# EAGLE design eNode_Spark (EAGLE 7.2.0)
REV: V3.3

## Sheet 1 of 4: Power & MCU
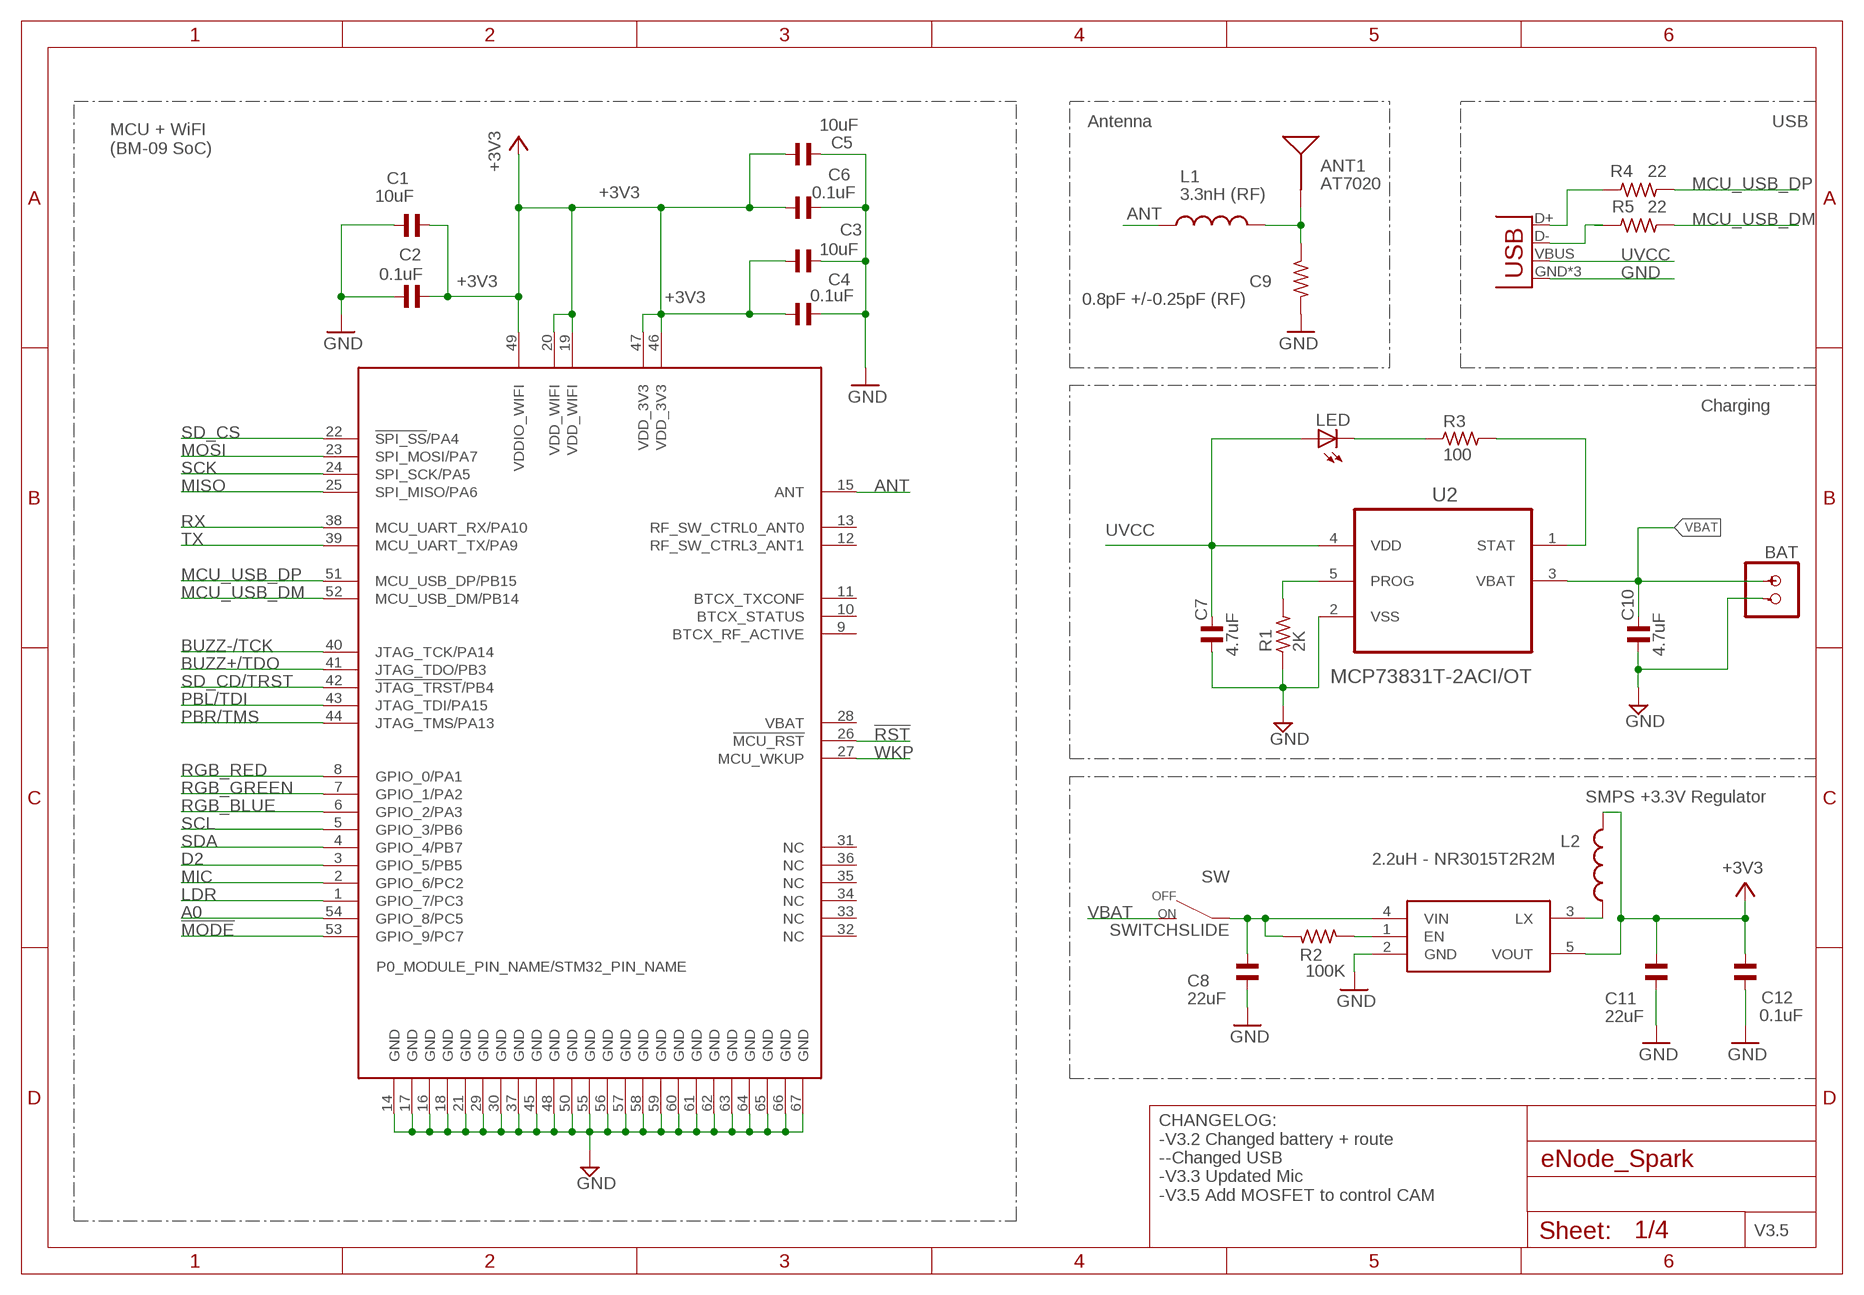
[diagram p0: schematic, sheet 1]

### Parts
ANT1  AT7020  [AT7020]
BAT  BATTERYSMT  [JST-2-SMD]
C1  10uF  C_0402  [C0402]
C2  0.1uF  C_0402  [C0402]
C3  10uF  C_0402  [C0402]
C4  0.1uF  C_0402  [C0402]
C5  10uF  C_0402  [C0402]
C6  0.1uF  C_0402  [C0402]
C7  4.7uF  C_0402  [C0402]
C8  22uF  C_0603  [C0603]
C9  0.8pF +/-0.25pF (RF)  R-US_  [R0402_B]
C10  4.7uF  C_0402  [C0402]
C11  22uF  C_0603  [C0603]
C12  0.1uF  C_0402  [C0402]
JP1  USBUSB-MICROB-SLOT-HOLE  [USB-MICROB-SLOT-HOLE]
L1  3.3nH (RF)  INDUCTOR  [L0402_B]
L2  2.2uH - NR3015T2R2M  INDUCTORB  [INDUCTOR-NR3015]
LED  LED  [SMARTLED-TTW]
R1  2K  R_0603  [R0603]
R2  100K  R_0402  [R0402]
R3  100  R_0603  [R0603]
R4  22  R_0402  [R0402]
R5  22  R_0402  [R0402]
SW  SWITCHSLIDE  [CHANGE_OVER_SLIDE]
U1  WM-N-BM-09  [WM-N-BM-09]
U2  MCP73831T-2ACI/OT  [SOT95P280X145-5N]
U3  R8008-33  [SOT23-5]

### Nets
!MODE: U1.53(GPIO_9/PC7) ; also sheet 3
!RST: U1.26(!MCU_RST) ; also sheet 3
+3V3: C1.2 C2.2 C3.1 C4.2 C5.1 C6.2 C11.1 C12.1 L2.2 U1.19(VDD_WIFI) U1.20(VDD_WIFI) U1.46(VDD_3V3) U1.47(VDD_3V3) U1.49(VDDIO_WIFI) U3.5(VOUT) ; also sheet 2,3,4
A0: U1.54(GPIO_8/PC5)
ANT [RF]: L1.1 U1.15(ANT)
BUZZ+/TDO: U1.41(JTAG_TDO/PB3) ; also sheet 3
BUZZ-/TCK: U1.40(JTAG_TCK/PA14) ; also sheet 3
D2: U1.3(GPIO_5/PB5) ; also sheet 4
ENABLE [vcc]: R2.1 U3.1(EN)
GND: BAT.- C1.1 C2.1 C3.2 C4.1 C5.2 C6.1 C7.1 C8.2 C9.2 C10.1 C11.2 C12.2 JP1.GND JP1.MT1(GND) JP1.MT2(GND) R1.1 U1.14(GND) U1.16(GND) U1.17(GND) U1.18(GND) U1.21(GND) U1.29(GND) U1.30(GND) U1.37(GND) U1.45(GND) U1.48(GND) U1.50(GND) U1.55(GND) U1.56(GND) U1.57(GND) U1.58(GND) U1.59(GND) U1.60(GND) U1.61(GND) U1.62(GND) U1.63(GND) U1.64(GND) U1.65(GND) U1.66(GND) U1.67(GND) U2.2(VSS) U3.2(GND) ; also sheet 2,3,4
LDR: U1.1(GPIO_7/PC3) ; also sheet 3
MCU_USB_DM: R5.1 U1.52(MCU_USB_DM/PB14)
MCU_USB_DP: R4.1 U1.51(MCU_USB_DP/PB15)
MF: JP1.D+ R4.2
MIC: U1.2(GPIO_6/PC2) ; also sheet 3
MISO: U1.25(SPI_MISO/PA6) ; also sheet 3,4
MOSI: U1.23(SPI_MOSI/PA7) ; also sheet 3,4
N$1 [RF]: ANT1.1(SIGNAL) C9.1 L1.2
N$2: C8.1 R2.2 SW.1 U3.4(VIN)
N$3: L2.1 U3.3(LX)
N$4: R1.2 U2.5(PROG)
N$5: LED.C@1(C) R3.1
N$6: R3.2 U2.1(STAT)
N$18: JP1.D- R5.2
PBL/TDI: U1.43(JTAG_TDI/PA15) ; also sheet 3
PBR/TMS: U1.44(JTAG_TMS/PA13) ; also sheet 3
RGB_BLUE [vcc]: U1.6(GPIO_2/PA3) ; also sheet 3
RGB_GREEN: U1.7(GPIO_1/PA2) ; also sheet 3
RGB_RED: U1.8(GPIO_0/PA1) ; also sheet 3
RX: U1.38(MCU_UART_RX/PA10) ; also sheet 3
SCK: U1.24(SPI_SCK/PA5) ; also sheet 3,4
SCL: U1.5(GPIO_3/PB6) ; also sheet 2,4
SD_CD/TRST: U1.42(!JTAG_TRST!/PB4) ; also sheet 3
SD_CS: U1.22(!SPI_SS!/PA4) ; also sheet 3,4
SDA: U1.4(GPIO_4/PB7) ; also sheet 2,4
TX: U1.39(MCU_UART_TX/PA9) ; also sheet 3
UVCC: C7.2 JP1.VBUS LED.A@1(A) U2.4(VDD)
VBAT: BAT.+ C10.2 SW.2 U2.3(VBAT)
WKP: U1.27(MCU_WKUP) ; also sheet 2,4
Unconnected: U1.9(BTCX_RF_ACTIVE) U1.10(BTCX_STATUS) U1.11(BTCX_TXCONF) U1.12(RF_SW_CTRL3_ANT1) U1.13(RF_SW_CTRL0_ANT0) U1.28(VBAT) U1.31(NC) U1.32(NC) U1.33(NC) U1.34(NC) U1.35(NC) U1.36(NC)

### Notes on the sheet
- Antenna | USB
- MCU + WiFI
  (BM-09 SoC)
- Charging
- SMPS +3.3V Regulator
- CHANGELOG:
  -V3.2 Changed battery + route
  --Changed USB
  -V3.3 Updated Mic
  -V3.5 Add MOSFET to control CAM
- V3.5

## Sheet 2 of 4: I2C
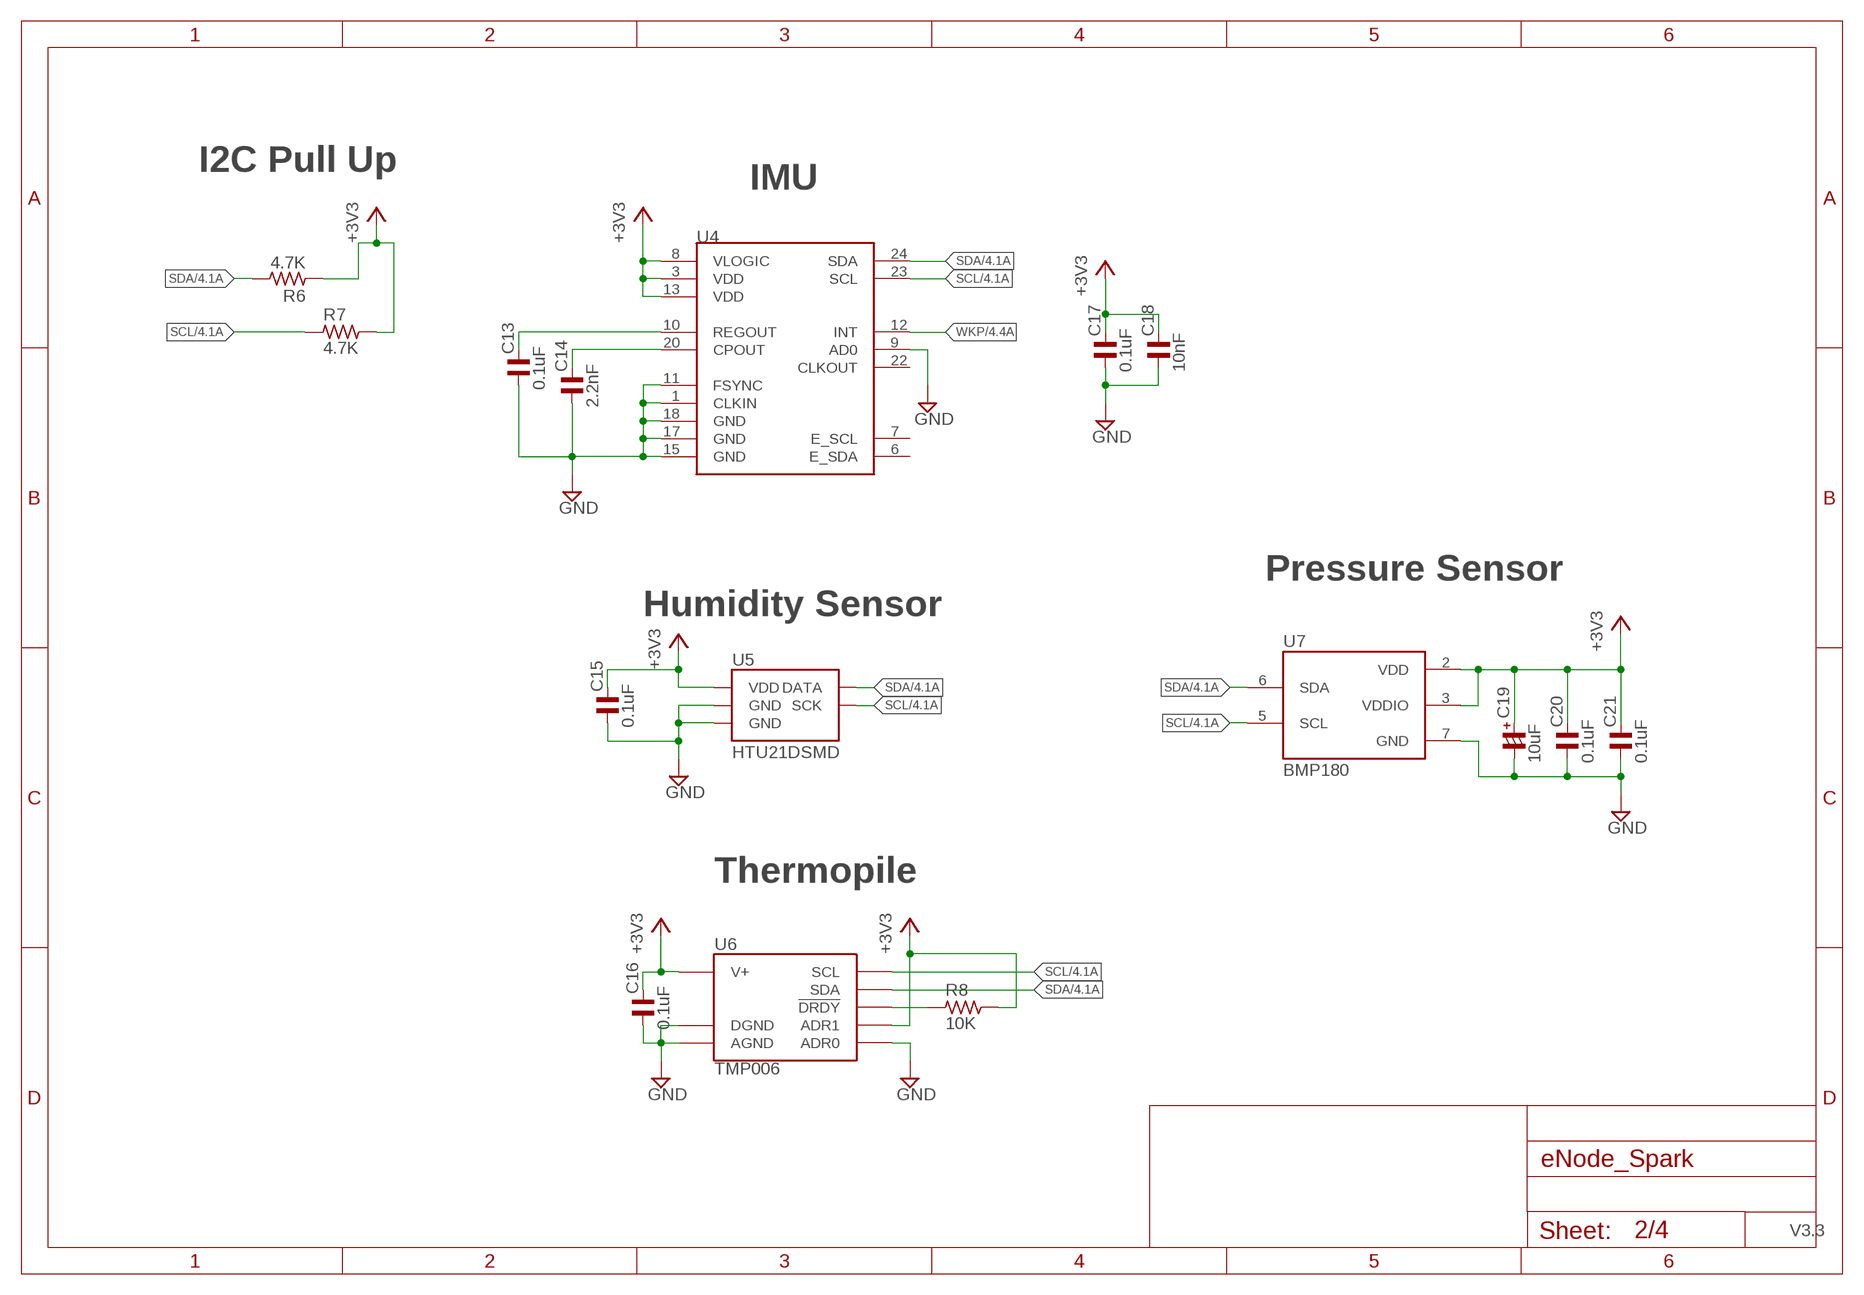
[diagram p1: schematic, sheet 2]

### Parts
C13  0.1uF  C_0402  [C0402]
C14  2.2nF  C_0402  [C0402]
C15  0.1uF  C_0402  [C0402]
C16  0.1uF  C_0402  [C0402]
C17  0.1uF  C_0402  [C0402]
C18  10nF  C_0402  [C0402]
C19  10uF  CP_1206/T  [C1206/T]
C20  0.1uF  C_0402  [C0402]
C21  0.1uF  C_0402  [C0402]
R6  4.7K  R_0402  [R0402]
R7  4.7K  R_0402  [R0402]
R8  10K  R_0603  [R0603]
U4  MPU-9150QFN-24-NP  [QFN-24-NP]
U5  HTU21DSMD  [HTU21D]
U6  TMP006  [BGA8DS]
U7  BMP180  [BMP180]

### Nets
+3V3: C15.2 C16.2 C17.2 C18.2 C19.+ C20.2 C21.2 R6.1 R7.2 R8.2 U4.3(VDD) U4.8(VLOGIC) U4.13(VDD) U5.VDD U6.A3(V+) U6.B1(ADR1) U7.2(VDD) U7.3(VDDIO) ; also sheet 1,3,4
GND: C13.1 C14.1 C15.1 C16.1 C17.1 C18.1 C19.- C20.1 C21.1 U4.1(CLKIN) U4.9(AD0) U4.11(FSYNC) U4.15(GND) U4.17(GND) U4.18(GND) U5.7(GND) U5.GND U6.A1(DGND) U6.A2(AGND) U6.C1(ADR0) U7.7(GND) ; also sheet 1,3,4
N$12: C14.2 U4.20(CPOUT)
N$13: R8.1 U6.C2(!DRDY)
N$14: C13.2 U4.10(REGOUT)
SCL: R7.1 U4.23(SCL) U5.SCK U6.B3(SCL) U7.5(SCL) ; also sheet 1,4
SDA: R6.2 U4.24(SDA) U5.DATA U6.C3(SDA) U7.6(SDA) ; also sheet 1,4
WKP: U4.12(INT) ; also sheet 1,4
Unconnected: U4.6(E_SDA) U4.7(E_SCL) U4.22(CLKOUT)

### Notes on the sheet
- I2C Pull Up
- IMU
- Pressure Sensor
- Humidity Sensor
- Thermopile

## Sheet 3 of 4: Other IO
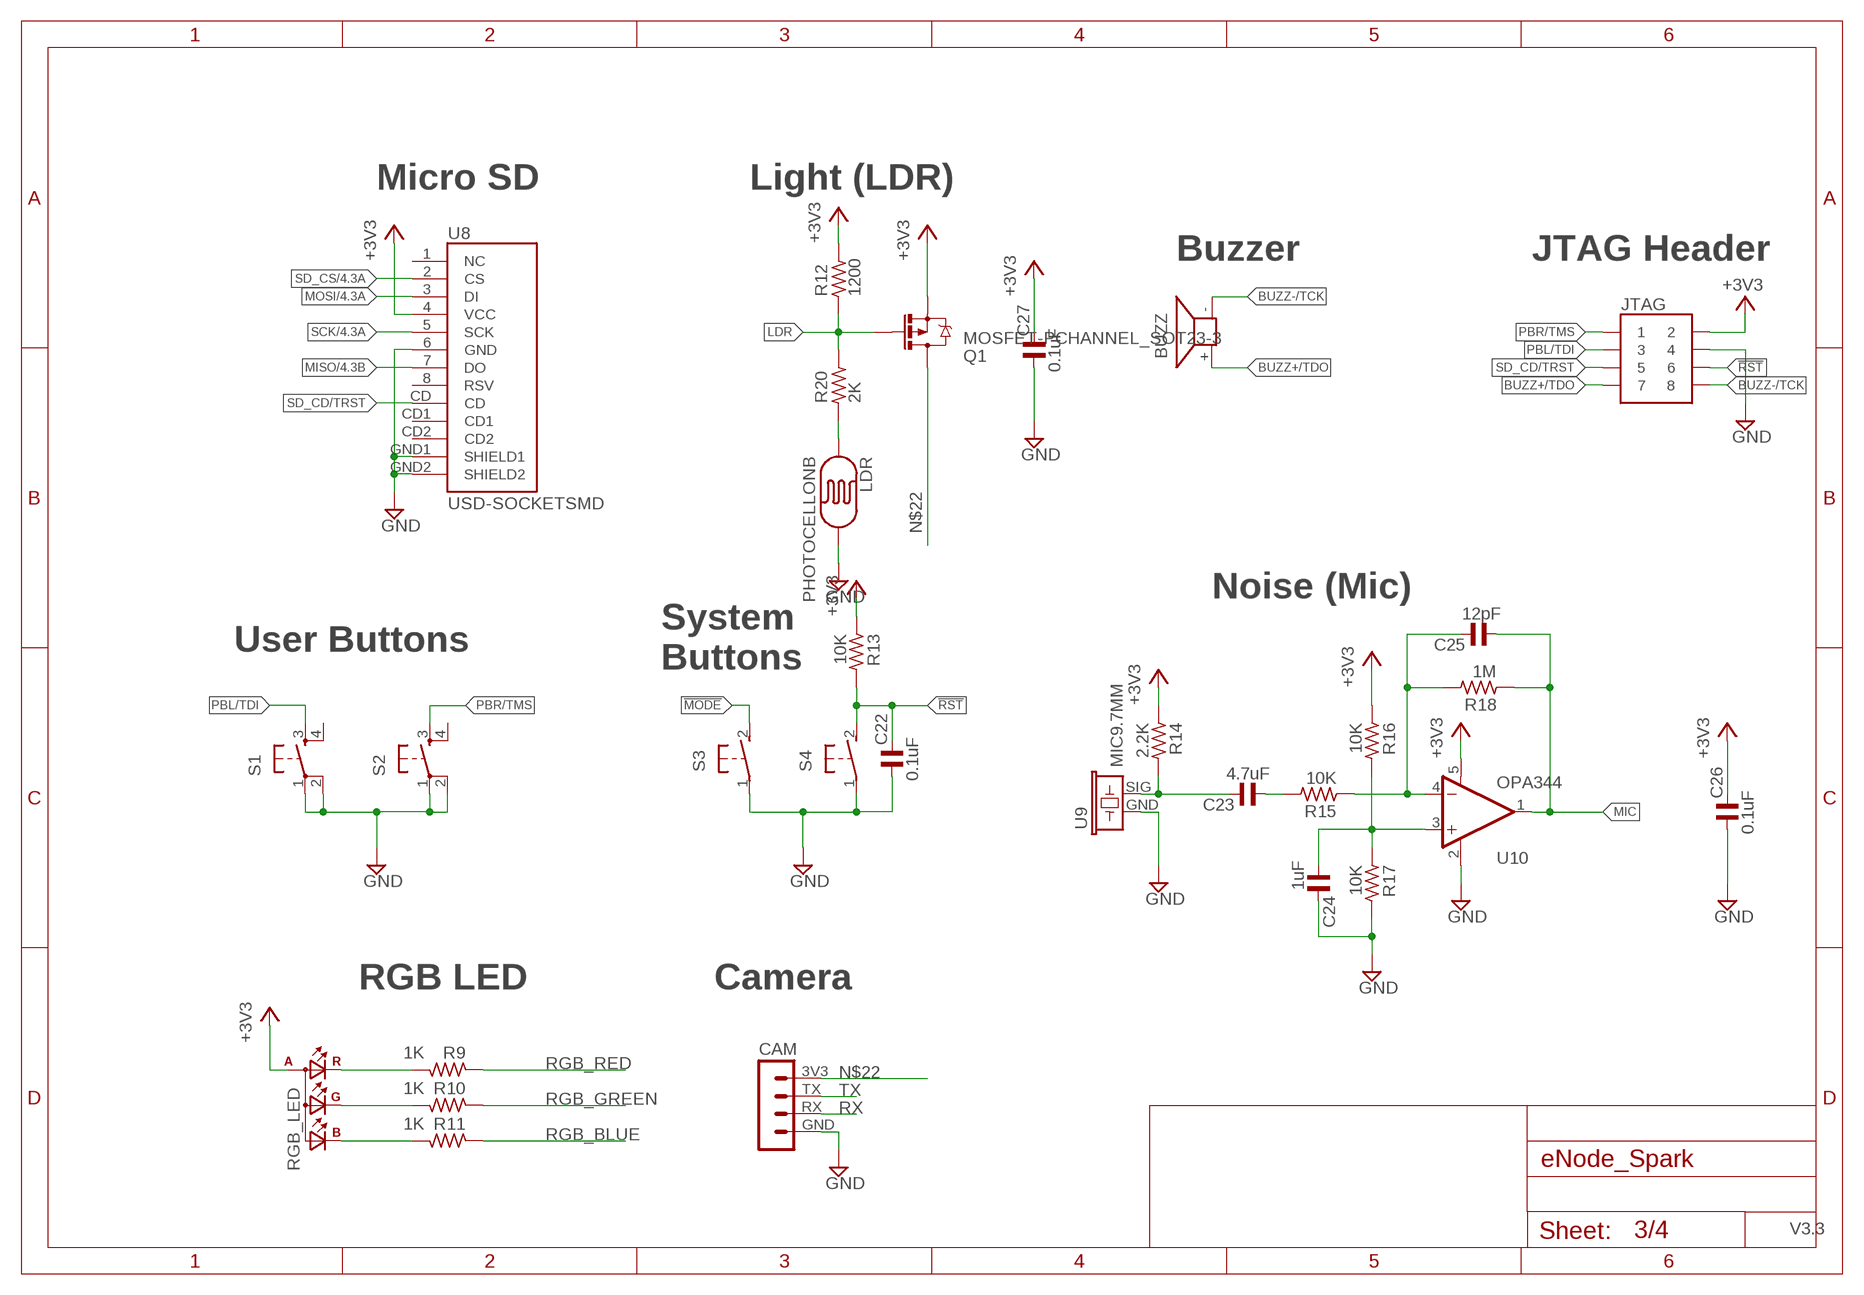
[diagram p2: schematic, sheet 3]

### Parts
BUZZ  BUZZER  [OFFBOARD_NOSIGN]
C22  0.1uF  C_0402  [C0402]
C23  4.7uF  C_0402  [C0402]
C24  1uF  C_0402  [C0402]
C25  12pF  C_0402  [C0402]
C26  0.1uF  C_0402  [C0402]
C27  0.1uF  C_0402  [C0402]
CAM  MA04-1  [MA04-1]
JTAG  JTAG_CONNECTOR  [JTAG_DIP]
LDR  PHOTOCELLONB  [ON_BOARD]
Q1  MOSFET-PCHANNEL_SOT23-3  [SOT23-3]
R9  1K  R_0402  [R0402]
R10  1K  R_0402  [R0402]
R11  1K  R_0402  [R0402]
R12  1200  R_0603  [R0603]
R13  10K  R_0402  [R0402]
R14  2.2K  R_0402  [R0402]
R15  10K  R_0402  [R0402]
R16  10K  R_0402  [R0402]
R17  10K  R_0402  [R0402]
R18  1M  R_0402  [R0402]
R20  2K  R_0603  [R0603]
RGB_LED  TOPLED-3PLCC  [P-LCC-4-3]
S1  TAC_SWITCH_4SMD  [TACTILE_SWITCH_SMD_LARGE_4]
S2  TAC_SWITCH_4SMD  [TACTILE_SWITCH_SMD_LARGE_4]
S3  MODE  TAC_SWITCH_2MULTICOMP  [DTSM-3]
S4  RESET  TAC_SWITCH_2MULTICOMP  [DTSM-3]
U8  USD-SOCKETSMD  [MICRO-SD-SOCKET-PP]
U9  MIC9.7MM  [MIC-9.7MM]
U10  OPA344  [SOT23-5]

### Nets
!MODE: S3.2 ; also sheet 1
!RST: C22.2 JTAG.6 R13.2 S4.2 ; also sheet 1
+3V3: C26.2 C27.2 JTAG.2 Q1.2(S) R12.2 R13.1 R14.1 R16.1 RGB_LED.A(A2) U8.4(VCC) U10.5(V+) ; also sheet 1,2,4
BUZZ+/TDO: BUZZ.+ JTAG.7 ; also sheet 1
BUZZ-/TCK: BUZZ.- JTAG.8 ; also sheet 1
GND: C22.1 C24.2 C26.1 C27.1 CAM.GND JTAG.4 LDR.2 R17.2 S1.1 S1.2 S2.1 S2.2 S3.1 S4.1 U8.6(GND) U8.GND1(SHIELD1) U8.GND2(SHIELD2) U9.GND U10.2(V-) ; also sheet 1,2,4
LDR: Q1.1(G) R12.1 R20.2 ; also sheet 1
MIC: C25.1 R18.1 U10.1(OUT) ; also sheet 1
MISO: U8.7(DO) ; also sheet 1,4
MOSI: U8.3(DI) ; also sheet 1,4
N$7: C23.1 R15.2
N$8: C25.2 R15.1 R18.2 U10.4(-IN)
N$9: C24.1 R16.2 R17.1 U10.3(+IN)
N$10: C23.2 R14.2 U9.SIG
N$11: LDR.1 R20.1
N$22: CAM.3V3 Q1.3(D)
N$27: R10.1 RGB_LED.G(CGREEN)
N$29: R11.1 RGB_LED.B(CBLUE)
N$54: R9.1 RGB_LED.R(CRED)
PBL/TDI: JTAG.3 S1.3 ; also sheet 1
PBR/TMS: JTAG.1 S2.3 ; also sheet 1
RGB_BLUE [vcc]: R11.2 ; also sheet 1
RGB_GREEN: R10.2 ; also sheet 1
RGB_RED: R9.2 ; also sheet 1
RX: CAM.RX ; also sheet 1
SCK: U8.5(SCK) ; also sheet 1,4
SD_CD/TRST: JTAG.5 U8.CD ; also sheet 1
SD_CS: U8.2(CS) ; also sheet 1,4
TX: CAM.TX ; also sheet 1
Unconnected: S1.4 S2.4 U8.1(NC) U8.8(RSV) U8.CD1 U8.CD2

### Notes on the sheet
- Micro SD | Light (LDR)
- Buzzer | JTAG Header
- Noise (Mic)
- User Buttons
- System
  Buttons
- RGB LED | Camera

## Sheet 4 of 4: V3.4
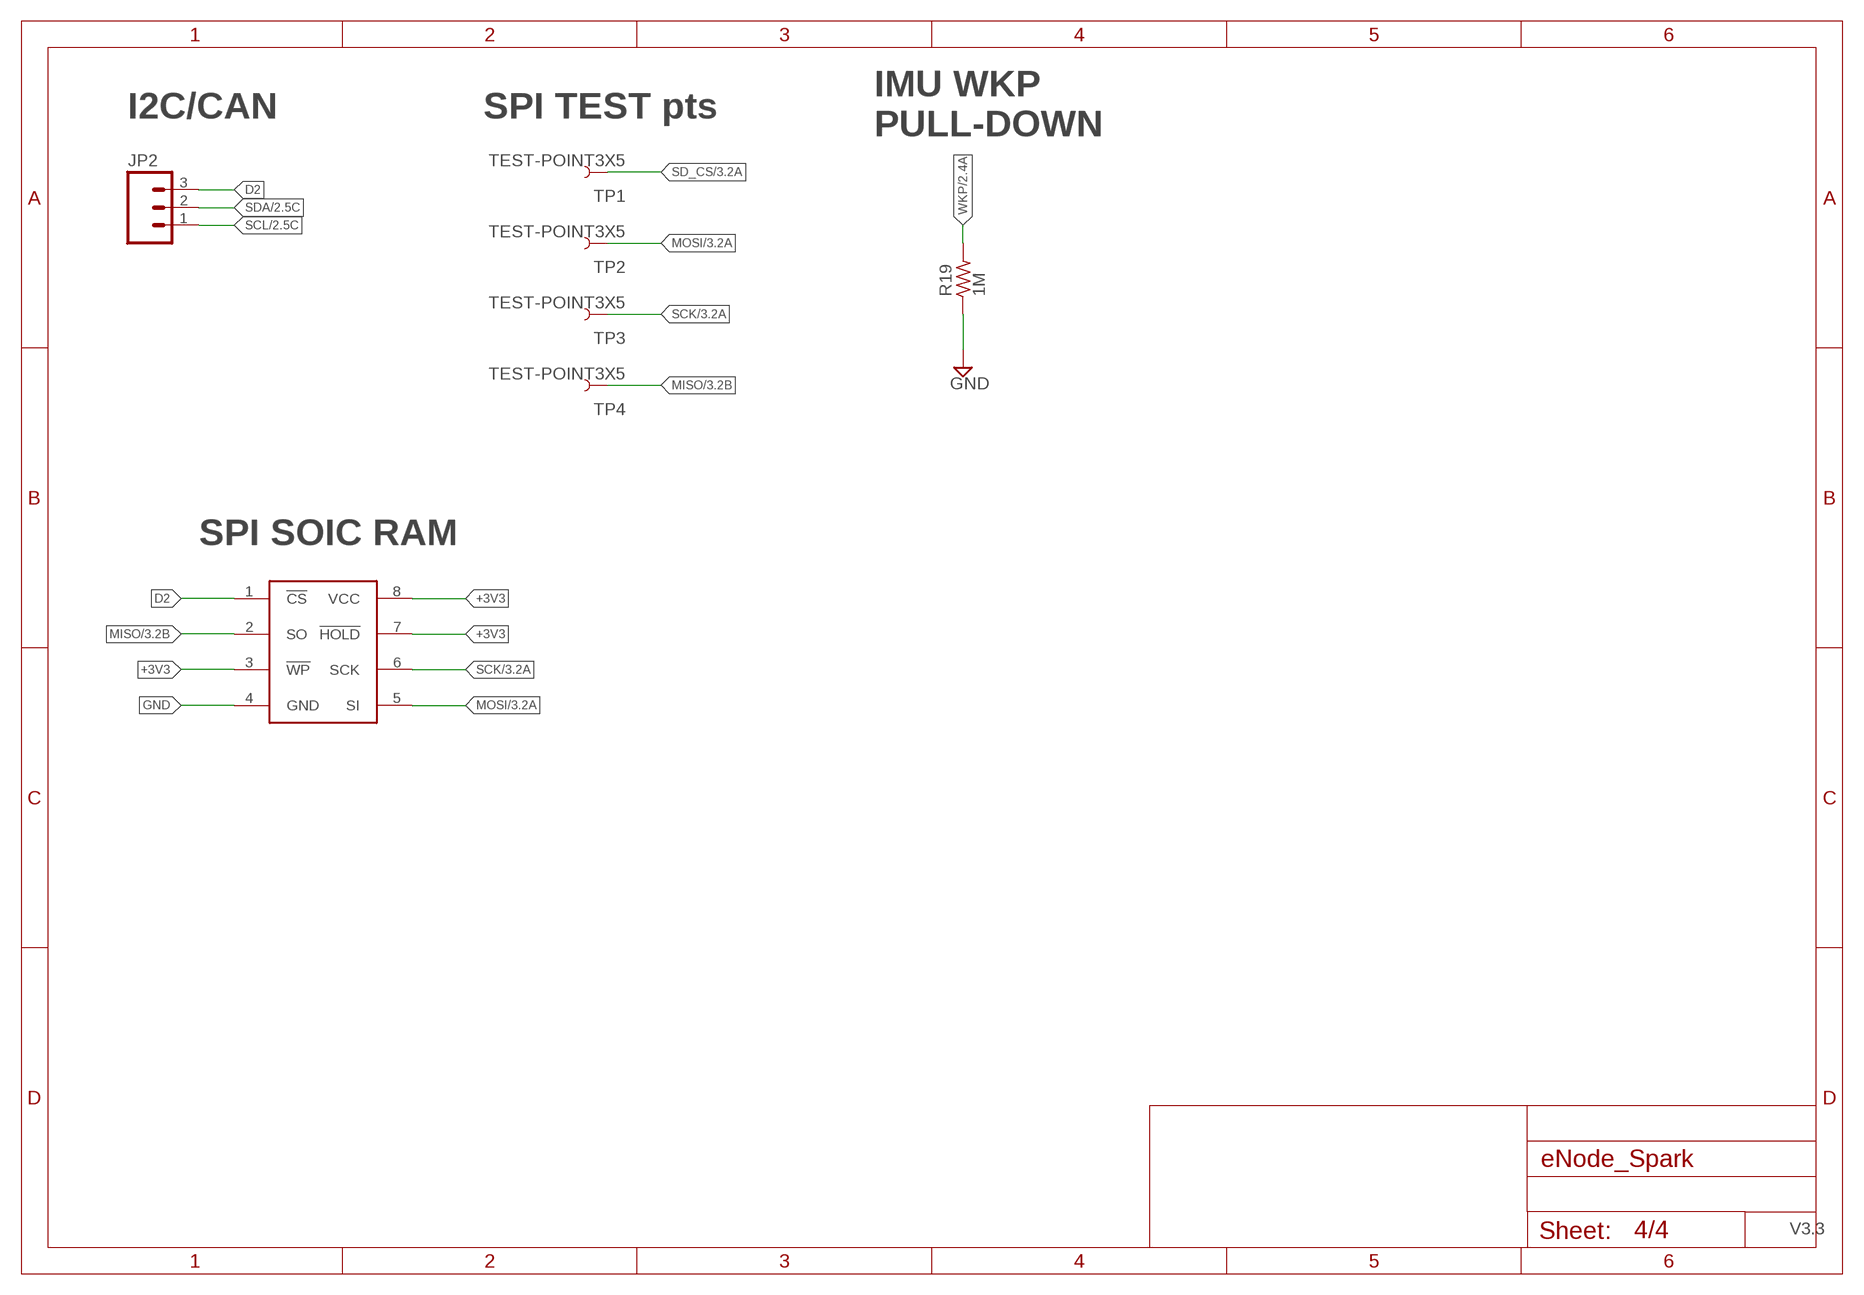
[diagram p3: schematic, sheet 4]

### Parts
JP2  M03PTH  [1X03]
R19  1M  R_0402  [R0402]
TP1  TEST-POINT3X5  [PAD.03X.05]
TP2  TEST-POINT3X5  [PAD.03X.05]
TP3  TEST-POINT3X5  [PAD.03X.05]
TP4  TEST-POINT3X5  [PAD.03X.05]
U11  FRAM  [SO08]

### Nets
+3V3: U11.3(!WP) U11.7(!HOLD) U11.8(VCC) ; also sheet 1,2,3
D2: JP2.3 U11.1(!CS) ; also sheet 1
GND: R19.1 U11.4(GND) ; also sheet 1,2,3
MISO: TP4.P$1 U11.2(SO) ; also sheet 1,3
MOSI: TP2.P$1 U11.5(SI) ; also sheet 1,3
SCK: TP3.P$1 U11.6(SCK) ; also sheet 1,3
SCL: JP2.1 ; also sheet 1,2
SD_CS: TP1.P$1 ; also sheet 1,3
SDA: JP2.2 ; also sheet 1,2
WKP: R19.2 ; also sheet 1,2

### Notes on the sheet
- I2C/CAN | SPI TEST pts
- IMU WKP 
  PULL-DOWN
- SPI SOIC RAM

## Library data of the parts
ANT1 = Spark:AT7020
BAT = Battery:BATTERY: PIN HEADER
BUZZ = Buzzer:BUZZER: Buzzer
C1-C8 C10-C18 C20-C27 = rc-master-smd:C_: NON-POLARIZED CAP
C9 = Spark:R-US_: 0402 Resistor
C19 = rc-master-smd:CP_: POLARIZED CAP
CAM = Camera Header:MA04-1: PIN HEADER; OC_FARNELL: unknown; OC_NEWARK: unknown
JP1 = Spark:USB
JP2 = SparkFun-Connectors:M03: Header 3 Standard 3-pin 0.1" header. Use with straight break away headers (SKU : PRT-00116), right angle break away headers (PRT-00553), swiss pins (PRT-00743), machine pins (PRT-00117), and female headers (PRT-00115). Molex polarized connector foot print use with SKU : PRT-08232 with associated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
JTAG = JTAG Connector:JTAG_CONNECTOR
L1 L2 = Spark:INDUCTOR
LDR = LDR:PHOTOCELL: Photo Resitor
LED = LED:LED: LED
Q1 = Simplex-DiscreteSemi:MOSFET-PCHANNEL: Generic P-channel mosfet
R1-R20 = rc-master-smd:R_: RESISTOR
RGB_LED = SMD RGB LED:TOPLED-3: Cree P/N: CLV1L-FKB-CHMMQEHBB7673673
S1 S2 = TACT BUTTON:TAC_SWITCH_4
S3 S4 = TACT BUTTON:TAC_SWITCH_2
SW = Switch:SWITCH
TP1-TP4 = SparkFun-Passives:TEST-POINT: Bare copper test points for troubleshooting or ICT
U1 = Spark:WM-N-BM-09
U2 = MCP73831T (LiPo Charger):MCP73831T-2ACI/OT: Charge Management Controller; MPN: MCP73831T-2ACI/OT; OC_FARNELL: 1332158; OC_NEWARK: 56K7045; PACKAGE: SOT-5; SUPPLIER: Microchip
U3 = Spark:R8008-33
U4 = MPU-9150:MPU-9150: 9DOF (3mag, 3accel, 3rotat). I2C interface.
U5 = HTU21D:HTU21D
U6 = TMP006:TMP006
U7 = BMP180:BMP180: BOSCH BMP180 DIGITAL BAROMETRIC PRESSURE SENSOR Web page: http://www.bosch-sensortec.com/en/homepage/products_3/environmental_sensors_1/bmp180_1/bmp180 Datasheet: http://ae-bst.resource.bosch.com/media/products/dokumente/bmp180/BST-BMP180-DS000-09.pdf The BMP180 is the function compatible successor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
U8 = MicroSD:USD-SOCKET: microSD Socket Push-push type uSD socket. Schematic element and footprint production proven. Spark Fun Electronics SKU : PRT-00127. tDoc lines correctly indicate media card edge positions when inserting (unlocked, locked, depressed).; ORDERCODE: 2143377; SUPPLIER: ELEMENT14
U9 = MIC:MIC: Microphone
U10 = OPA344:OPA344
U11 = kennethlimcp:FRAM: 8-SOIC FRAM

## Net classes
2 RF: width 0.33 mm, clearance 0.178 mm

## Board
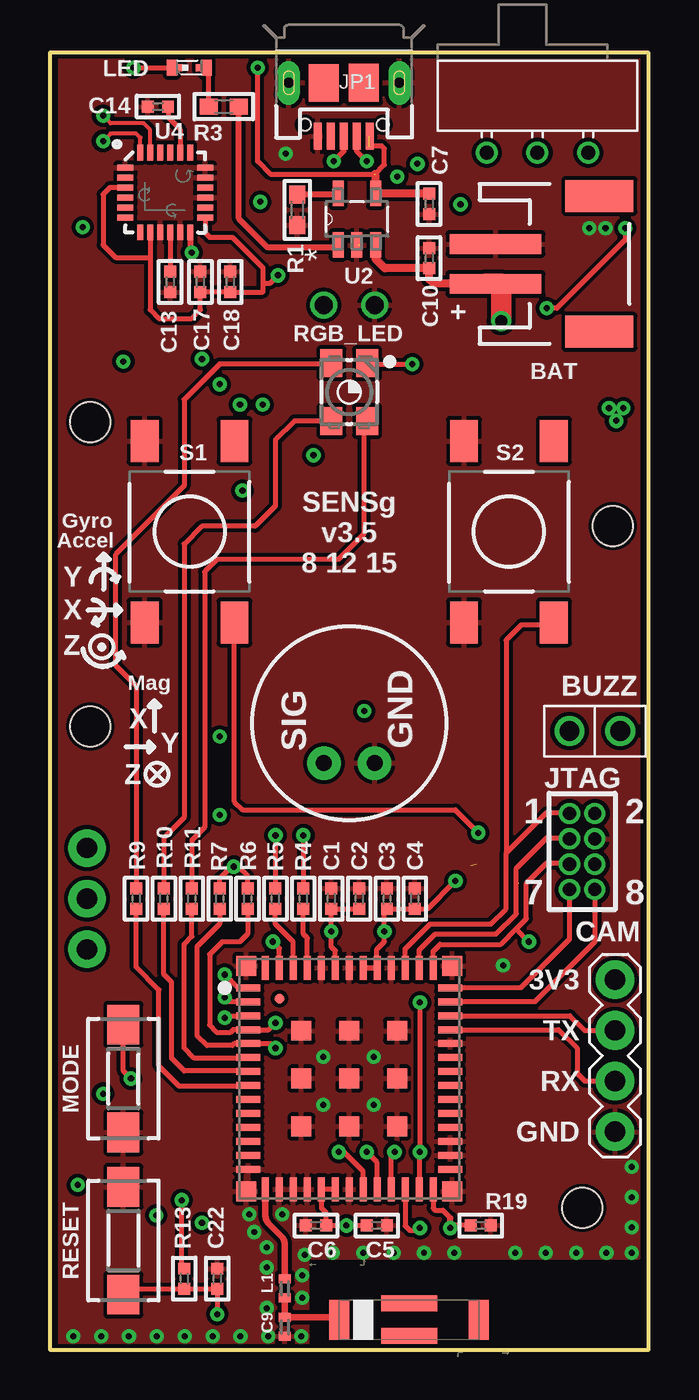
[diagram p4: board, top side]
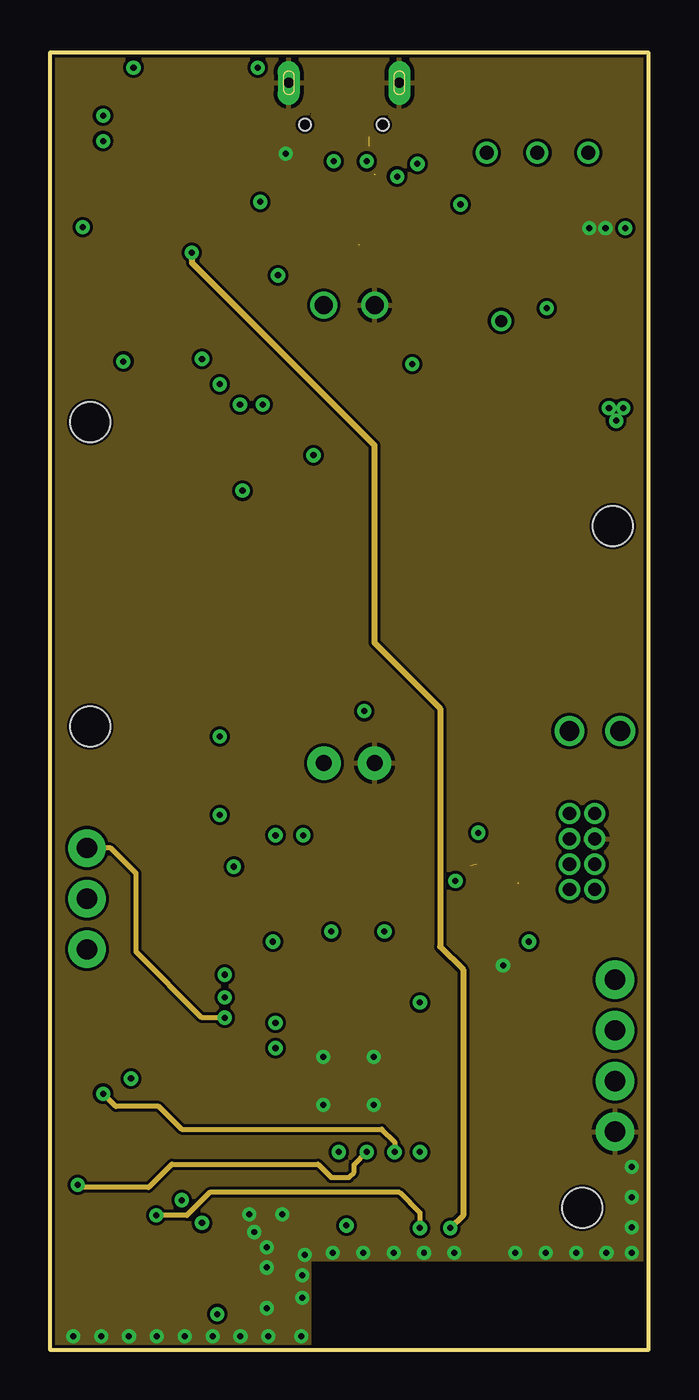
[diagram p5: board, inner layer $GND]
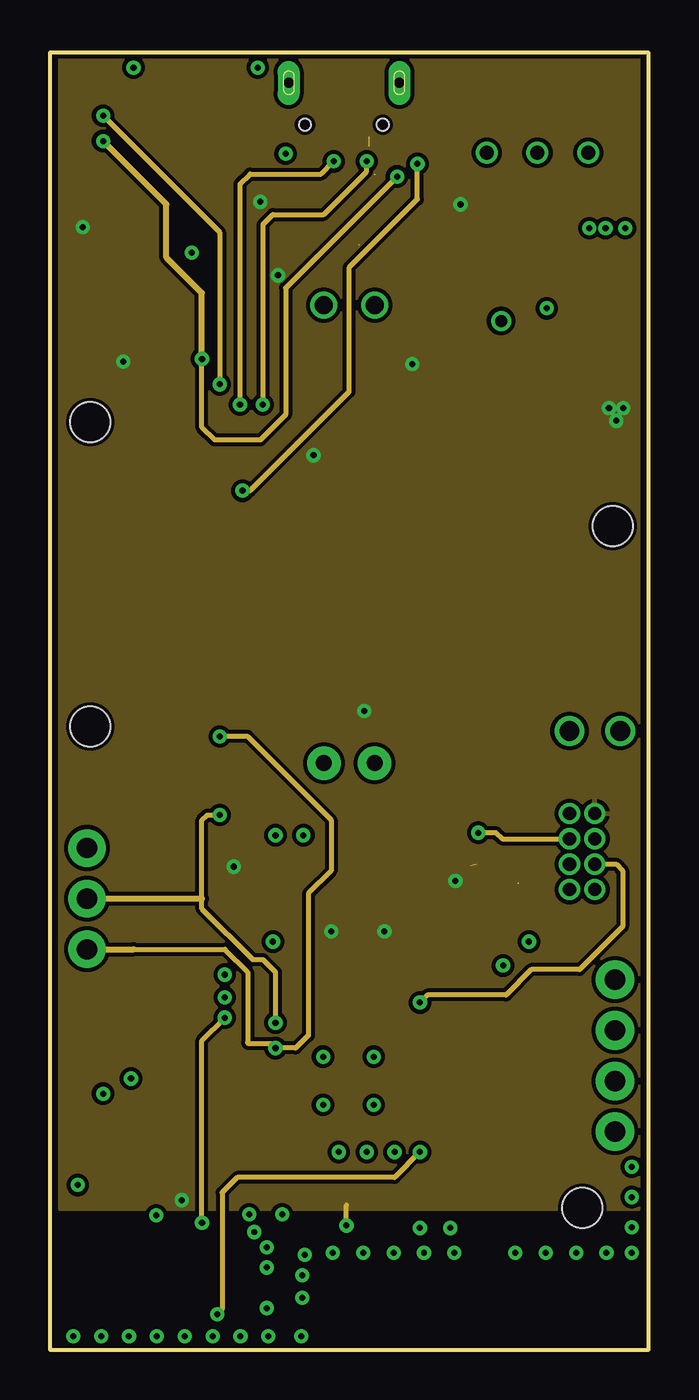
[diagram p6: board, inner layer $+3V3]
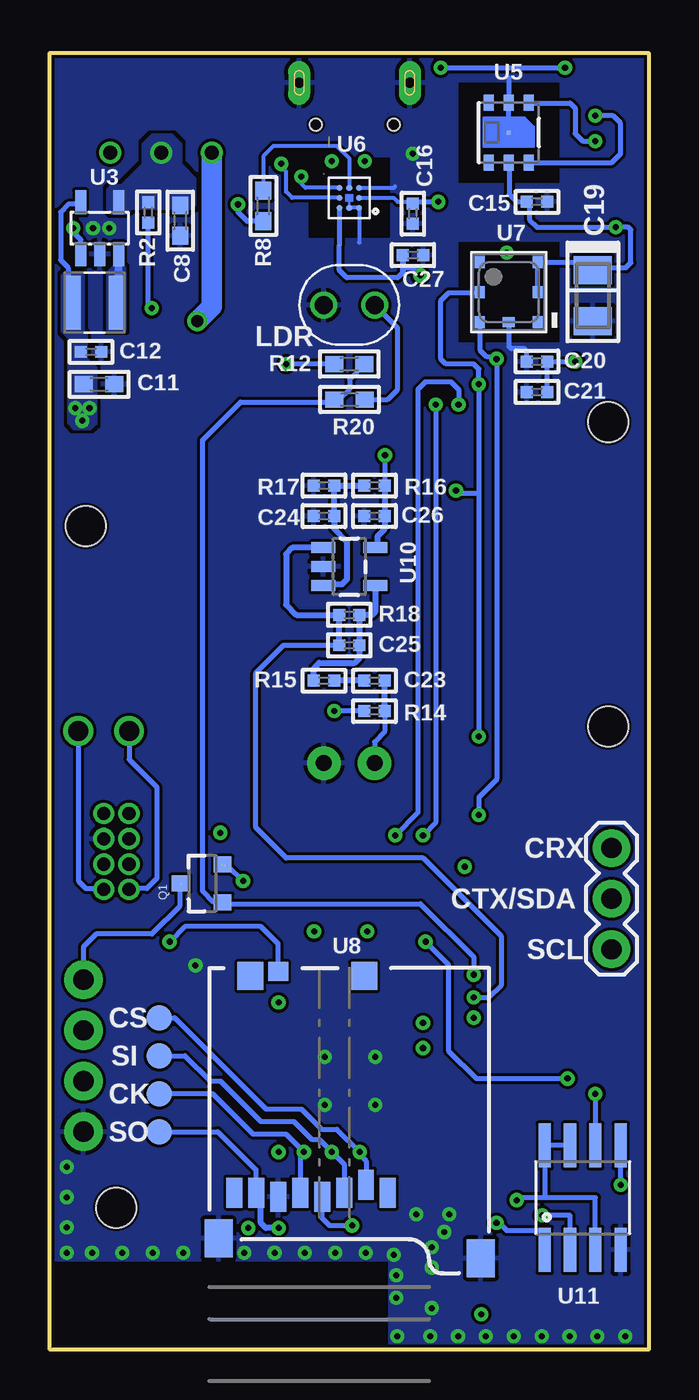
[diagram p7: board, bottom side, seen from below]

Size 30 x 65 mm. Coordinates in mm from the lower left corner, seen from the top.
Outline: 0,0 30,0 30,65 0,65 0,0
Copper layers (1+2*15+16): Top 0.018mm / dielectric 0.195mm / $GND 0.035mm / dielectric 1.1mm / $+3V3 0.035mm / dielectric 0.195mm / Bottom 0.018mm
Design rules "spark-4layer-custom": minimum track width 6mil, minimum drill 0.3mm, track to track 6mil, track to pad 6mil, pad to pad 6mil, via to via 6mil, smd to smd 6mil, copper to edge 6mil, drill to drill 6mil, minimum pad ring 8mil, minimum via ring 8mil, stop-mask expansion 4mil, vias tented up to drill 20mil, thermal gap 8mil
Holes 2 mm at 26.67,7.11 28.19,41.27 2.03,46.48 2.03,31.24

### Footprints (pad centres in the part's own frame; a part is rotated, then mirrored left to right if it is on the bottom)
AT7020 = smd 1 x 2: 1 3.5,0; 3 -3.5,0 | smd 2.8 x 0.8: 2 0,0.815; 4 0,-0.815
JST-2-SMD = smd 1 x 4.6: + 1,-3.7; - -1,-3.7 | smd 1.6 x 3.4: NC1 -3.4,1.5; NC2 3.4,1.5
OFFBOARD_NOSIGN = drill 1: + -1.27,0; - 1.27,0
C0402 = smd 0.6 x 0.6: 1 -0.508,0; 2 0.508,0
C0603 = smd 0.9 x 0.8: 1 -0.762,0; 2 0.762,0
R0402_B = smd 0.457 x 0.61: 1 -0.483,0; 2 0.483,0
C1206/T = smd 1.4 x 1.9: + 1.27,0; - -1.27,0
MA04-1 = drill 1.016 pad 1.93: 3V3 3.81,0; GND -3.81,0; RX -1.27,0; TX 1.27,0
USB-MICROB-SLOT-HOLE = smd 0.4 x 1.35: D+ 0,2.675; D- -0.65,2.675; GND 1.3,2.675; ID 0.65,2.675; VBUS -1.3,2.675 | drill 0.5 pad 1.1 long: MT1 -2.775,0; MT2 2.775,0 | smd 1.5 x 1.9: P$1 -1,0; P$2 1,0.01 | hole 0.6: -1.95,2.1; 1.95,2.1
1X03 = drill 1.016 pad 1.88: 1 0,0; 2 2.54,0; 3 5.08,0
JTAG_DIP = drill 0.66 pad 1.016: 1 0,0; 2 1.27,0; 3 0,-1.27; 4 1.27,-1.27; 5 0,-2.54; 6 1.27,-2.54; 7 0,-3.81; 8 1.27,-3.81
L0402_B = smd 0.457 x 0.61: 1 -0.483,0; 2 0.483,0
INDUCTOR-NR3015 = smd 0.8 x 2.7: 1 -1.1,0; 2 1.1,0
ON_BOARD = drill 0.9: 1 -1.27,0; 2 1.27,0
SMARTLED-TTW = smd 0.8 x 0.5: A 0,-0.875; C 0,0.875 | smd 0.35 x 0.35: A@1 0,-0.5; C@1 0,0.5
SOT23-3 = smd 0.8 x 0.9: 1 -0.95,-1; 2 0.95,-1; 3 0,1.1
R0603 = smd 0.9 x 0.8: 1 -0.762,0; 2 0.762,0
R0402 = smd 0.6 x 0.6: 1 -0.508,0; 2 0.508,0
P-LCC-4-3 = smd 1.1 x 1.4: A 0.9,1.45; B 0.9,-1.45; G -0.9,-1.45; R -0.9,1.45
TACTILE_SWITCH_SMD_LARGE_4 = smd 1.4 x 2.1: 1 2.25,4.55; 2 2.25,-4.55; 3 -2.25,4.55; 4 -2.25,-4.55
DTSM-3 = smd 2 x 1.6: 1 -2.7,0; 2 2.7,0
CHANGE_OVER_SLIDE = drill 0.7: 1 0,0; 2 -2.54,0; 3 2.54,0
PAD.03X.05 = smd 1.27 x 1.27: P$1 0,0
WM-N-BM-09 = smd 0.35 x 1.2: 1 4.55,5.05; 2 3.85,5.05; 3 3.15,5.05; 4 2.45,5.05; 5 1.75,5.05; 6 1.05,5.05; 7 0.35,5.05; 8 -0.35,5.05; 9 -1.05,5.05; 10 -1.75,5.05; 11 -2.45,5.05; 12 -3.15,5.05; 13 -3.85,5.05; 14 -4.55,5.05; 28 -4.55,-5.05; 29 -3.85,-5.05; 30 -3.15,-5.05; 31 -2.45,-5.05; 32 -1.75,-5.05; 33 -1.05,-5.05; 34 -0.35,-5.05; 35 0.35,-5.05; 36 1.05,-5.05; 37 1.75,-5.05; 38 2.45,-5.05; 39 3.15,-5.05; 40 3.85,-5.05; 41 4.55,-5.05 | smd 1.2 x 0.35: 15 -5.55,4.2; 16 -5.55,3.5; 17 -5.55,2.8; 18 -5.55,2.1; 19 -5.55,1.4; 20 -5.55,0.7; 21 -5.55,0; 22 -5.55,-0.7; 23 -5.55,-1.4; 24 -5.55,-2.1; 25 -5.55,-2.8; 26 -5.55,-3.5; 27 -5.55,-4.2; 42 5.55,-4.2; 43 5.55,-3.5; 44 5.55,-2.8; 45 5.55,-2.1; 46 5.55,-1.4; 47 5.55,-0.7; 48 5.55,0; 49 5.55,0.7; 50 5.55,1.4; 51 5.55,2.1; 52 5.55,2.8; 53 5.55,3.5; 54 5.55,4.2 | smd 1 x 1: 55 5.65,5.15; 56 -5.65,5.15; 57 -5.65,-5.15; 58 5.65,-5.15; 59 2.4,2.4; 60 0,2.4; 61 -2.4,2.4; 62 2.4,0; 63 0,0; 64 -2.4,0; 65 2.4,-2.4; 66 0,-2.4; 67 -2.4,-2.4 | smd 0.5 x 0.5: 68 4,3.5
SOT95P280X145-5N = smd 1.27 x 0.559: 1 -1.295,0.94; 2 -1.295,0; 3 -1.295,-0.94; 4 1.295,-0.94; 5 1.295,0.94
SOT23-5 = smd 0.55 x 1.2: 1 -0.95,-1.3; 2 0,-1.3; 3 0.95,-1.3; 4 0.95,1.3; 5 -0.95,1.3
QFN-24-NP = smd 0.8 x 0.3: 1 -2,1.25; 2 -2,0.75; 3 -2,0.25; 4 -2,-0.25; 5 -2,-0.75; 6 -2,-1.25; 13 2,-1.25; 14 2,-0.75; 15 2,-0.25; 16 2,0.25; 17 2,0.75; 18 2,1.25 | smd 0.3 x 0.8: 7 -1.25,-2; 8 -0.75,-2; 9 -0.25,-2; 10 0.25,-2; 11 0.75,-2; 12 1.25,-2; 19 1.25,2; 20 0.75,2; 21 0.25,2; 22 -0.25,2; 23 -0.75,2; 24 -1.25,2
HTU21D = smd 0.2 x 0.2: 7 0,0 | smd 0.8 x 0.5: DATA 1.5,-1; GND 1.5,0; NC@1 -1.5,1; NC@6 1.5,1; SCK -1.5,-1; VDD -1.5,0
BGA8DS = smd 0.305 x 0.305: A1 0.5,-0.5; A2 0,-0.5; A3 -0.5,-0.5; B1 0.5,0; B3 -0.5,0; C1 0.5,0.5; C2 0,0.5; C3 -0.5,0.5
BMP180 = smd 0.6 x 0.5: 1 1.5,1.45; 2 0,1.45; 3 -1.5,1.45; 4 -1.5,-1.45; 5 0,-1.45; 6 1.5,-1.45 | smd 0.5 x 0.6: 7 1.5,0
MICRO-SD-SOCKET-PP = smd 0.8 x 1.5: 1 7.54,-11.26; 2 6.44,-10.86; 3 5.34,-11.26; 4 4.24,-11.46; 5 3.14,-11.26; 6 2.04,-11.46; 7 0.94,-11.26; 8 -0.16,-11.26 | smd 1 x 0.95: CD 2.04,-0.175 | smd 1.3 x 1.4: CD1 6.35,-0.4; CD2 0.65,-0.4 | smd 1.4 x 1.9: GND1 12.2,-14.55; GND2 -0.95,-13.55
MIC-9.7MM = drill 0.8 pad 1.676: GND -2,-1.27; SIG -2,1.27
SO08 = smd 0.61 x 2.21: 1 -1.905,-2.616; 2 -0.635,-2.616; 3 0.635,-2.616; 4 1.905,-2.616; 5 1.905,2.616; 6 0.635,2.616; 7 -0.635,2.616; 8 -1.905,2.616

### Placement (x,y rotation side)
ANT1  18,1.5 180 top
BAT  26.03,54.42 270 top
BUZZ  27.3,31 0 top
C1  14.1,22.61 270 top
C2  15.49,22.61 270 top
C3  16.89,22.61 90 top
C4  18.29,22.61 270 top
C5  16.38,6.22 0 top
C6  13.34,6.22 0 top
C7  19,57.43 90 top
C8  23.47,56.59 270 bottom
C9  11.77,1.14 270 top
C10  19,54.71 270 top
C11  27.53,48.39 0 bottom
C12  27.94,50.01 0 bottom
C13  6.02,53.52 90 top
C14  5.41,62.31 0 top
C15  5.59,57.53 180 bottom
C16  11.81,56.94 90 bottom
C17  7.54,53.52 270 top
C18  9.04,53.52 270 top
C19  2.79,52.83 90 bottom
C20  5.59,49.53 0 bottom
C21  5.59,48.01 0 bottom
C22  8.38,3.56 270 top
C23  13.73,33.53 0 bottom
C24  16.27,41.78 180 bottom
C25  15,35.31 0 bottom
C26  13.73,41.78 0 bottom
C27  11.81,54.86 180 bottom
CAM  28.32,14.73 90 top
JP1  14.73,63.5 180 top
JP2  1.85,20.07 90 bottom
JTAG  26.04,26.87 0 top
L1  11.77,3.07 270 top
L2  27.76,52.48 180 bottom
LDR  15,52.37 180 bottom
LED  6.99,64.26 270 top
Q1  22.35,23.37 90 bottom
R1  12.4,57.12 90 top
R2  25.07,57 90 bottom
R3  8.71,62.31 0 top
R4  12.7,22.61 90 top
R5  11.3,22.61 90 top
R6  9.91,22.61 270 top
R7  8.51,22.61 90 top
R8  19.3,57.32 270 bottom
R9  4.32,22.61 270 top
R10  5.71,22.61 270 top
R11  7.11,22.61 270 top
R12  15,49.4 180 bottom
R13  6.73,3.56 270 top
R14  13.73,32 0 bottom
R15  16.27,33.53 0 bottom
R16  13.73,43.31 180 bottom
R17  16.27,43.31 180 bottom
R18  15,36.83 0 bottom
R19  21.59,6.22 180 top
R20  14.99,47.62 180 bottom
RGB_LED  15,48 0 top
S1  7,41 180 top
S2  23,41 180 top
S3  3.68,13.59 90 top
S4  3.68,5.46 270 top
SW  24.43,60 0 top
TP1  24.51,16.64 0 bottom
TP2  24.51,14.73 0 bottom
TP3  24.51,12.83 0 bottom
TP4  24.51,10.92 0 bottom
U1  15,13.59 90 top
U2  15.38,56.67 90 top
U3  27.51,56.21 0 bottom
U4  5.78,58 0 top
U5  7,61 90 bottom
U6  15,57.74 0 bottom
U7  7,53 270 bottom
U8  20.6,19.13 0 bottom
U9  15,31.4 90 top
U10  15,39.24 270 bottom
U11  3.3,7.62 0 bottom

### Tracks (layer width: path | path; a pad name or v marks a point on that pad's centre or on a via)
!MODE  (via drill 0.3)
  Top 0.254: U1.53 11.5,20.12 v11.18,20.45 | v4.06,13.59 3.68,13.97 S3.2
  Bottom 0.254: v11.18,20.45 10.03,19.3 10.03,14.99 8.64,13.59 v4.06,13.59
!RST  (via drill 0.3, 0.3 pad 0.3)
  Top 0.254: U1.26 18.5,9.91 v18.54,9.91 v18.54,17.4 | S4.2 3.97,3.05 R13.2 C22.2 v8.38,1.78
  $+3V3 0.254: JTAG.6 28.37,24.33 28.7,24 28.7,21.21 26.54,19.05 24.13,19.05 22.86,17.78 18.92,17.78 v18.54,17.4 | v18.54,9.91 17.27,8.64 9.4,8.64 8.64,7.87 8.64,2.03 v8.38,1.78
+3V3  (via drill 0.3)  (2 unrouted)
  Top 0.254: U1.46 U1.47 16.34,19.14 16.38,19.18 16.38,20.07 16.76,20.45 v16.76,20.95 16.76,21.97 C3.1 C4.2 18.92,22.1 v20.32,23.5 | RGB_LED.A 15.95,49.4 v18.16,49.4 | R13.1 6.6,4.19 v6.6,7.49 | C5.1 v14.86,6.22 C6.2 13.84,6.86 13.6,7.1 U1.19 U1.20 | 15.37,22.1 C2.2 C1.2 v14.1,20.95 14.1,20.19 14.3,19.99 U1.49 | R6.1 9.91,23.75 9.45,24.21 v9.22,24.21 9.09,24.21 8.51,23.62 R7.2 | U4.13 7.78,55.98 8,55.75 9.14,55.75 10.67,54.23 10.67,53.47 | U4.8 5.03,54.74 | 5.03,54.74 5.03,52.12 5.46,51.69 7.11,51.69 7.54,52.12 C17.2 C18.2 10.67,53.01 10.67,53.47 | U4.3 3,58.25 2.67,57.91 2.67,55.37 3.3,54.74 5.03,54.74 | 10.67,53.47 11.05,53.47 v11.43,53.85
  $+3V3 0.254: v14.86,6.22 14.86,7.24
  Bottom 0.203: U6.B1 12.78,57.74 12.57,57.53 11.89,57.53 C16.2
  Bottom 0.254: 2.92,54.23 C19.+ 2.67,54.23 | U7.2 U7.3 3.19,54.5 2.92,54.23 | v3.68,49.53 C20.2 C21.2 | U5.VDD 6.99,59.48 6.99,57.91 6.6,57.53 C15.2 5.97,57.4 5.97,56.64 5.59,56.26 v1.65,56.26 1.02,56.26 0.89,56.13 0.89,54.48 1.14,54.23 2.92,54.23 | C16.2 11.73,57.53 v10.54,57.53 | U6.A3 15.5,55.38 | 28.57,57.4 29.08,57.4 29.46,57.02 29.46,54.61 29.08,54.23 29.08,52.7 L2.2 | R16.1 13.21,43.32 v13.21,44.83 | U8.4 16.38,7.65 16.38,6.6 16,6.22 v14.86,6.22 | R14.1 v15.75,32 | R8.2 20.11,56.56 20.57,57.02 v20.57,57.4 | U11.7 U11.8 5.21,7.62 | U11.3 2.67,7.62 5.21,7.62 | 5.21,7.62 6.48,7.62 v6.6,7.49 | 21.08,24.26 v20.32,23.5 | 12.32,53.98 12.57,53.72 15.11,53.72 15.49,54.1 15.49,55.37 | 12.32,54.23 11.81,54.23 v11.43,53.85 | R12.2 v18.16,49.4
  Bottom 0.305: R16.1 C26.2 13.22,41.13 13.59,40.77 13.59,40.3 U10.5 | C27.2 12.32,54.23 12.32,53.98
  Bottom 0.406: U3.5 28.57,57.51 28.57,57.4
  other vias: 28.02,47.19 28.73,47.19 28.37,46.56
  pour Bottom (no thermals): 28.3,53.9 28.42,54.05 29.24,54.05 29.46,53.85 29.46,51.03 29.13,50.7 29.13,46.43 28.8,46.1 27.97,46.1 27.64,46.38 27.64,49.25 28.09,49.71 28.09,50.88 28.24,51.05 28.24,53.85
  pour $+3V3 (isolate 0.203, rank 2): 0.5,65 29.5,65 29.5,7 0.5,7
ANT
  Top 0.33: L1.1 11.77,5.24 arc45 11.59,5.68 10.99,6.29 arc-45 10.8,6.74 U1.15
BUZZ+/TDO
  Top 0.254: JTAG.7 26.04,20.57 23.6,18.14 U1.41
  Bottom 0.254: BUZZ.+ 26.04,29.59 24.64,28.19 24.64,23.62 25.15,23.11 25.98,23.11 JTAG.7
BUZZ-/TCK
  Top 0.254: JTAG.8 27.3,20.45 24.3,17.44 U1.40
  Bottom 0.254: BUZZ.- 28.57,23.5 28.19,23.11 27.36,23.11 JTAG.8
D2  (via drill 0.3, 0.3 pad 0.71)
  Top 0.254: v8.76,16.64 8.87,16.74 U1.3
  $GND 0.254: v8.76,16.64 7.62,16.64 4.32,19.94 4.32,23.88 3.05,25.15 JP2.3
  $+3V3 0.254: v7.62,6.35 7.62,15.49 v8.76,16.64
  Bottom 0.254: U11.1 5.21,5.71 5.46,5.97 7.11,5.97 7.49,6.35 v7.62,6.35
ENABLE  (via drill 0.3)
  Top 0.254: v28.83,56.21 28.83,55.63 25.4,52.2 v24.89,52.2
  Bottom 0.254: U3.1 28.45,54.92 28.45,55.63 28.83,56.01 v28.83,56.21 | v24.89,52.2 25.07,52.38 R2.1
GND  (via drill 0.3)
  Bottom 0.203: U6.C1 12.76,58.24 12.7,58.29 | 14.48,55.5 14.5,55.5 U6.A1 U6.A2
  Bottom 0.254: U7.7 7,50.29 6.87,50.16 6.22,50.16 6.1,50.04 C20.1 | 6.99,63.75 6.99,62.52 U5.GND U5.7
  other vias: 27.03,56.21 27.84,56.21 16.23,14.68 13.69,14.68 13.69,12.27 16.23,12.27 22.71,19.25 12.6,0.66 10.95,0.66 12.65,2.59 12.65,3.73 12.78,4.75 14.17,4.85 15.7,4.85 17.22,4.85 18.75,4.85 20.27,4.85 23.32,4.85 24.84,4.85 26.37,4.85 27.89,4.85 29.16,4.85 29.16,6.12 29.16,7.65 29.16,9.17 9.55,0.66 8.15,0.66 6.76,0.66 3.96,0.66 5.36,0.66 2.57,0.66 1.17,0.66 11.63,6.78 9.98,6.78 10.24,5.89 10.87,5.13 10.87,4.11 10.87,2.08 11.81,59.94
  pour $GND: 0,65 30,65 30,4.5 13,4.5 13,0 0,0
  pour Top (isolate 0.203, rank 3): 0.5,65 29.5,65 29.5,4.58 12.92,4.58 12.92,0 0.5,0
  pour Bottom (rank 2): 0,65 30,65 30,4.5 13,4.5 13,0 0,0
LDR  (via drill 0.3)
  Top 0.254: v8.76,18.8 9.4,18.16 9.93,18.16 U1.1
  Bottom 0.254: v8.76,18.8 8.76,19.68 11.43,22.35 21.29,22.35 Q1.1 21.78,22.42 22.35,22.99 22.35,45.59 20.45,47.5 15.88,47.5 R20.2 | R20.2 15.73,47.62 | R12.1 14.99,48.66 14.99,48.13 15.49,47.62 R20.2
MCU_USB_DM
  Top 0.254: U1.52 12.19,20.45 11.3,21.34 R5.1
MCU_USB_DP
  Top 0.254: U1.51 12.9,20.63 12.7,20.83 R4.1
MF  (via drill 0.3)
  Top 0.254: v12.7,25.78 R4.2 | v14.22,59.56 14.73,60.07 JP1.D+
  $+3V3 0.254: v9.53,47.37 9.53,58.42 10.03,58.93 13.59,58.93 v14.22,59.56
  Bottom 0.254: v12.7,25.78 11.56,26.92 11.56,48.13 11.18,48.51 9.91,48.51 9.53,48.13 v9.53,47.37
MIC  (via drill 0.3)
  Top 0.254: U1.2 8.98,17.44 v8.76,17.65
  Bottom 0.254: C25.1 18.29,35.31 19.68,33.91 19.68,26.16 18.16,24.64 11.3,24.64 7.37,20.7 7.37,18.29 8,17.65 v8.76,17.65
  Bottom 0.305: C25.1 R18.1 17.65,36.83 18.16,37.34 18.16,39.88 17.85,40.19 U10.1
MISO  (via drill 0.3, 0.3 pad 0.71)
  Top 0.254: U1.25 17.8,6.2 18.03,5.97 18.41,5.97 v18.54,6.1
  $GND 0.254: v5.33,6.73 6.86,6.73 8,7.87 17.53,7.87 18.54,6.86 v18.54,6.1
  Bottom 0.254: TP4.P$1 21.59,10.92 19.68,9.02 19.68,7.89 U8.7 | U11.2 3.94,6.73 v5.33,6.73
  Bottom 0.305: v18.54,6.1 19.18,6.1 19.43,6.35 19.43,7.64 U8.7
MOSI  (via drill 0.3)
  Top 0.254: U1.23 16.4,9.38 v15.88,9.91
  $GND 0.254: v1.4,8.26 1.52,8.13 4.95,8.13 6.12,9.29 13.44,9.29 14.1,8.64 14.99,8.64 15.24,8.89 15.24,9.27 v15.88,9.91
  Bottom 0.254: U8.3 15.26,9.29 v15.88,9.91 16.51,10.54 16.89,10.54 17.78,11.43 19.43,11.43 21.46,13.46 21.97,13.46 23.24,14.73 TP2.P$1 | v1.4,8.26 U11.5
N$1
  Top 0.33: L1.2 C9.1 14.37,1.63 ANT1.1
N$2
  pour Bottom (isolate 0.254, no thermals): 23.37,59.44 23.37,60.45 23.88,60.96 24.89,60.96 25.4,60.45 25.4,59.44 26.42,58.42 26.92,58.42 27.18,58.17 27.18,57.15 26.92,56.9 26.16,56.9 25.91,57.15 22.86,57.15 22.61,57.4 22.61,58.67
N$3
  Bottom 0.406: L2.1 26.56,52.58 U3.3
  pour Bottom (no thermals): 26.26,54.33 26.16,54.23 26.16,51.1 26.24,51.03 27.1,51.03 27.18,51.1 27.18,53.85 27.18,54 26.85,54.33
N$4
  Top 0.305: U2.5 14.37,57.89 R1.2
N$5
  Top 0.254: 8,62.36 R3.1 7.95,64.26 LED.C@1
N$6
  Top 0.305: U2.1 14.31,55.24 10.92,55.24 9.47,56.69 R3.2
N$7
  Bottom 0.305: C23.1 R15.2
N$8
  Bottom 0.305: U10.4 13.7,36.97 13.84,36.83 R18.2 C25.2 14.48,35.29 14.48,34.67 14.73,34.42 16.51,34.42 16.78,34.15 R15.1
N$9
  Bottom 0.305: R16.2 R17.1 C24.1 15.76,41.16 15.11,40.51 15.11,38.61 15.37,38.35 16.24,38.35 U10.3
N$10
  Bottom 0.254: R14.2 13.22,30.97 13.73,30.47 U9.SIG
  Bottom 0.305: R14.2 C23.2
N$11
  Bottom 0.254: R20.1 13.08,47.62 12.57,48.13 12.57,51.21 LDR.1
N$12
  Top 0.254: C14.2 5.92,61.77 6.53,61.16 U4.20
N$13
  Bottom 0.203: U6.C2 14.99,58.25 14.99,59.69 15.62,60.33 18.8,60.33 19.3,59.82 R8.1
N$14
  Top 0.254: U4.10 C13.2
N$15
  cutout $GND: 13.05,61.96 13.06,61.96 arc-91
N$16
  cutout $GND: 16.95,61.96 16.96,61.96 arc-91
N$18  (via drill 0.3)
  Top 0.254: v11.3,25.78 R5.2 | v15.88,59.56 15.38,60.06 JP1.D-
  $+3V3 0.254: v10.67,47.37 10.67,56.39 11.18,56.9 13.72,56.9 15.88,59.05 v15.88,59.56
  Bottom 0.254: v10.67,47.37 10.67,26.42 v11.3,25.78
N$20
  cutout Bottom: 13.05,61.96 13.06,61.96 arc-91
N$21
  cutout Bottom: 16.95,61.96 16.96,61.96 arc-91
N$22  (1 unrouted)
  Bottom 0.254: 23.5,23.37 23.5,22.23 24.89,20.83 27.69,20.83 28.32,20.19 CAM.3V3
N$23
  cutout Bottom (no thermals): 13,59.74 13,55.74 17,55.74 17,59.74
  cutout Bottom (no thermals): 4.5,63.5 4.5,58.5 9.5,58.5 9.5,63.5
  cutout Bottom (no thermals): 4.5,55.5 4.5,50.5 9.5,50.5 9.5,55.5
N$27
  Top 0.254: RGB_LED.G 12.26,46.55 11.3,45.59 11.3,42.29 10.29,41.27 7.62,41.27 6.73,40.39 6.73,26.67 5.71,25.65 R10.1
N$29
  Top 0.254: RGB_LED.B 15.75,46.4 15.75,40.89 14.48,39.62 8.38,39.62 7.75,38.99 7.75,26.16 7.11,25.53 R11.1
N$54
  Top 0.254: RGB_LED.R 14.05,49.4 8.51,49.4 6.73,47.62 6.73,43.31 3.3,39.88 3.3,34.29 4.32,33.27 R9.1
PBL/TDI  (via drill 0.3)
  Top 0.254: U1.43 18.5,20.02 19.3,20.83 22.35,20.83 23.37,21.84 23.37,24.13 24.89,25.65 25.98,25.65 JTAG.3 | 8.76,35.96 S1.3 9.25,27.45 9.65,27.05 20.32,27.05 v21.46,25.91
  $+3V3 0.254: JTAG.3 22.66,25.6 22.35,25.91 v21.46,25.91
PBR/TMS
  Top 0.254: U1.44 17.8,20.09 19.05,21.34 22.1,21.34 22.86,22.1 22.86,24.38 22.86,24.89 | 22.86,24.89 24.89,26.92 25.98,26.92 JTAG.1 | S2.3 25.12,36.32 23.62,36.32 22.86,35.56 22.86,24.89
RGB_BLUE
  Top 0.254: U1.6 9.92,14.61 7.24,14.61 6.73,15.11 6.73,20.32 7.11,20.7 R11.2
RGB_GREEN
  Top 0.254: U1.7 9.92,13.97 6.73,13.97 6.1,14.61 6.1,18.41 5.71,18.8 R10.2
RGB_RED
  Top 0.254: U1.8 9.92,13.21 6.48,13.21 5.46,14.22 5.46,18.03 4.32,19.18 R9.2
RX
  Top 0.254: U1.38 25.49,16.04 26.42,15.11 26.42,13.84 26.8,13.46 CAM.RX
SCK  (via drill 0.3)
  Top 0.254: U1.24 17.1,9.73 v17.27,9.91
  $GND 0.254: v2.67,12.83 3.3,12.19 5.46,12.19 6.6,11.05 16.64,11.05 17.27,10.41 v17.27,9.91
  Bottom 0.254: v17.27,9.91 17.46,9.72 | 17.46,9.72 U8.5 | 17.46,9.72 17.46,10.09 18.16,10.79 19.81,10.79 21.84,12.83 TP3.P$1 | v2.67,12.83 U11.6
SCL  (via drill 0.3)
  Top 0.203: U4.23 5.03,61.14 4.7,61.47 3.05,61.47 v2.67,61.85
  Top 0.254: R7.1 8.51,21.34 7.37,20.19 7.37,15.75 7.87,15.24 9.14,15.24 9.24,15.34 U1.5 11.08,15.34 v11.3,15.11
  $+3V3 0.254: v2.67,61.85 8.51,56.01 v8.51,48.39 | v8.51,30.73 9.91,30.73 14.1,26.54 14.1,24 12.95,22.86 12.95,15.75 12.32,15.11 v11.3,15.11 11.08,15.34 U1.5 9.91,15.38 9.91,18.92 8.76,20.07 4.19,20.07 | v9.65,43.05 10.03,43.05 14.99,48.01 14.99,54.23 18.41,57.66 v18.41,59.44
  $+3V3 0.305: JP2.1 4.19,20.07
  Bottom 0.203: U6.B3 17.86,57.74 18.16,58.04 18.16,59.05 18.41,59.31 v18.41,59.44
  Bottom 0.254: U7.5 8.49,52.96 10.03,52.96 10.41,52.58 10.41,49.66 10.16,49.4 8.76,49.4 8.51,49.15 v8.51,48.39 8.51,42.93 | U5.SCK 1.84,59.5 1.4,59.94 1.4,61.47 1.78,61.85 v2.67,61.85 | 8.51,42.93 v8.51,30.73 | v9.65,43.05 9.53,42.93 8.51,42.93
SD_CD/TRST  (via drill 0.3)
  Top 0.254: U1.42 19.2,19.96 19.56,20.32 22.61,20.32 23.37,21.08 | 23.37,21.08 23.88,21.59 23.88,23.37 24.89,24.38 25.98,24.38 JTAG.5 | v24,20.45 23.37,21.08
  Bottom 0.254: U8.CD 18.56,20.34 19.43,21.21 23.24,21.21 v24,20.45
SD_CS  (via drill 0.3)
  Top 0.254: U1.22 15.7,8.94 14.73,9.91 v14.48,9.91
  Bottom 0.254: U8.2 14.16,9.46 14.48,9.78 v14.48,9.91 15.62,11.05 16.38,11.05 17.4,12.06 19.18,12.06 23.75,16.64 TP1.P$1
SDA  (via drill 0.3)
  Top 0.203: U4.24 4.53,60.75 4.32,60.96 3.05,60.96 v2.67,60.58
  Top 0.254: R6.2 9.91,20.83 9.53,20.45 8.64,20.45 8,19.81 8,16.26 8.35,15.91 9.05,15.91 9.18,16.04 U1.4 10.96,16.04 v11.3,16.38
  $+3V3 0.254: v8.51,26.8 7.87,26.8 7.62,26.54 7.62,22.61 7.62,22.1 10.16,19.56 10.67,19.56 11.3,18.92 v11.3,16.38 | v7.62,49.66 7.62,46.23 8.26,45.59 10.54,45.59 11.81,46.86 11.81,53.21 v17.4,58.8
  $+3V3 0.305: JP2.2 7.62,22.61 | 2.79,60.58 v2.67,60.58 5.84,57.4 5.84,54.74 7.62,52.96 v7.62,49.66
  Bottom 0.203: U6.C3 17.2,58.24 17.4,58.44 v17.4,58.8 | U5.DATA 5.98,62.48
  Bottom 0.254: 8.52,51.44 U7.6 8.45,50.11 8.13,49.78 7.75,49.78 v7.62,49.66 7.62,28.57 8.51,27.69 v8.51,26.8 | 5.98,62.48 3.94,62.48 3.68,62.23 3.68,60.96 3.3,60.58 v2.67,60.58
TX
  Top 0.254: U1.39 26.06,16.74 26.8,16 CAM.TX
UVCC  (via drill 0.3)  (2 unrouted)
  Top 0.254: v10.41,64.26 10.41,59.56 11.05,58.93 16.26,58.93 | JP1.VBUS 16,60.8 | 16.3,58.93 16.76,59.39 16.76,60.2 16.64,60.33 16,60.33 | v4.19,64.26 LED.A@1
  Top 0.406: C7.2 19,57.96 U2.4 16.3,57.96 16.3,58.93
  Bottom 0.254: v10.41,64.26 v4.19,64.26
VBAT  (via drill 0.6)
  Top 0.406: BAT.+ 21.84,53.42 19.22,53.42 19,53.65 C10.2 | 18.92,54.13 C10.2 | C10.2 16.79,54.2 16.32,54.67 U2.3
  Top 1.016: 21.84,53.42 22.61,53.42 v22.61,51.56
  Bottom 1.016: v22.61,51.56 21.89,52.28 SW.2
WKP  (via drill 0.3 pad 0.71)
  Top 0.254: U1.27 19.2,7.09 19.3,6.99 19.68,6.99 20.07,6.6 | R19.2 20.19,6.22 v20.07,6.1
  Top 0.305: U4.12 7.03,55.08 v7.11,54.99 | v20.07,6.1 20.07,6.6
  $GND 0.305: v7.11,54.99 7.11,54.48 16.26,45.34 16.26,35.43 19.56,32.13 19.56,20.19 20.7,19.05 20.7,6.73 v20.07,6.1

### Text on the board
tPlace: + | SENSg | Gyro | v3.5 | Accel | 8 12 15 | Y | X | Z | Mag | X | Y | Z | MODE | RESET
bNames: CRX | CTX/SDA | SCL | CS | SI | CK | SO
tDocu: NOTES: / / Layer stack up: / 1 - GTL - Top Copper / 2 - G2L - Inner Ground / 15 - G15L - Inner +3.3V / 16 - GBL - Bottom Copper | REV: | CHANGELOG: / -V3.2 Changed Battery "+" / Route / --Changed USB / --Removed Short / --Updated MIC / -V3.3 Corrected for DFM / Errors

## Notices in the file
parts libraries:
rc-master-smd: Copyright (C) 2007-2008, Bob Starr
SparkFun-Connectors: Licensing: Creative Commons ShareAlike 4.0 International - https://creativecommons.org/licenses/by-sa/4.0
